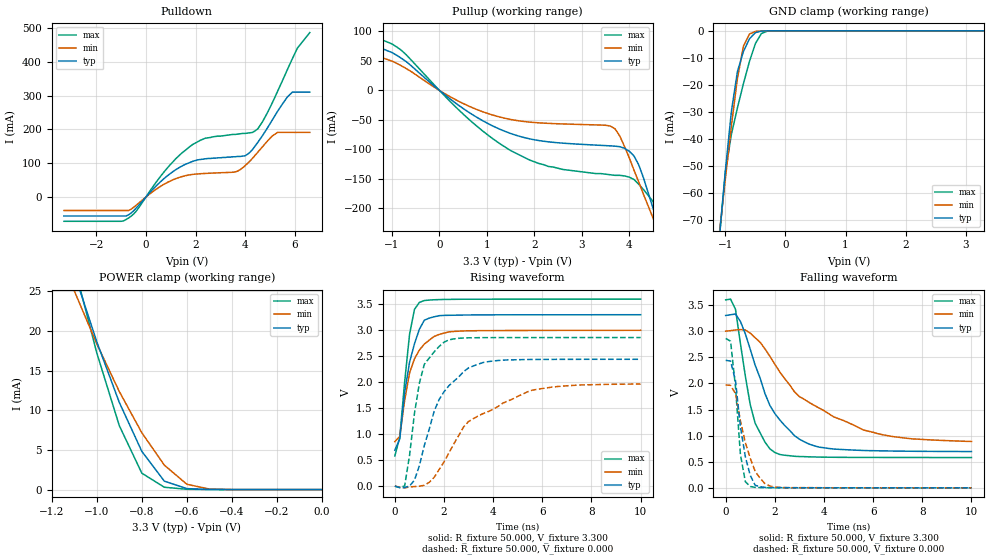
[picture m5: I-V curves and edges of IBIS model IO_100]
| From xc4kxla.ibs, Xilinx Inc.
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|   Model IO_100
[Model]   IO_100
Model_type   I/O
Polarity   Non-Inverting
Enable   Active-Low
Vinl =   0.800V
Vinh =   2.000V
Vmeas =   1.650V
Cref =  50.000pF
Rref =   1.000M
Vref =  0.000V
C_comp   7.300pF   5.500pF   8.800pF
[Temperature Range]   50.000   100.000   0.000
[Voltage Range]   3.300V   3.000V   3.600V
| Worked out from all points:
|   slope of the pulldown table from 0 to 0.495 V, typ, clamps not added: 12.8 ohm
|   slope of the pullup table from 0 to 0.495 V, typ, clamps not added: 16.3 ohm
|   GND clamp passes 1 mA (typ) near -0.52 V on its own axis
|   POWER clamp passes 1 mA (typ) near -0.69 V on its own axis
|   rising waveform, R_fixture 50.000, V_fixture 3.300: 20-80 % time 558ps typ, 647ps min, 383ps max; typ from 0.693 V to 3.3 V
|   rising waveform, R_fixture 50.000, V_fixture 0.000: 20-80 % time 1.2ns typ, 2.41ns min, 577ps max; typ from 0 V to 2.44 V
|   falling waveform, R_fixture 50.000, V_fixture 3.300: 20-80 % time 1.44ns typ, 2.95ns min, 729ps max; typ from 3.3 V to 0.696 V
|   falling waveform, R_fixture 50.000, V_fixture 0.000: 20-80 % time 438ps typ, 650ps min, 309ps max; typ from 2.44 V to 0.001 V
[Pulldown]
| voltage   I(typ)   I(min)   I(max)
-3.3V     -56.02mA   -39.74mA   -71.65mA
-900mV    -56.02mA   -39.74mA   -70.27mA
-400mV    -33.2mA    -24.66mA   -42.45mA
900mV     64.82mA    44.51mA    89.05mA
1.8V      103mA      66.09mA    151mA
3.6V      119mA      74.19mA    185mA
4V        122mA      93.03mA    188mA
4.5V      161mA      132mA      201mA
5.3V      253mA      191mA      312mA
5.7V      296mA      191mA      377mA
6.1V      310mA      191mA      440mA
6.6V      310mA      191mA      486mA
[Pullup]
| voltage   I(typ)   I(min)   I(max)
-3.3V     90.2mA     70.7mA     105mA
-1.9V     87mA       69.42mA    102mA
-1V       64.22mA    49.76mA    78.82mA
500mV     -30.67mA   -22.15mA   -40.1mA
1.5V      -72.97mA   -49.19mA   -102mA
2.3V      -87.2mA    -55.86mA   -129mA
3.6V      -94mA      -60.31mA   -143mA
3.8V      -95.43mA   -77.13mA   -144mA
4.1V      -111mA     -135mA     -151mA
4.5V      -199mA     -216mA     -188mA
4.7V      -250mA     -255mA     -227mA
6.6V      -645mA     -572mA     -737mA
[GND_clamp]
| voltage   I(typ)   I(min)   I(max)
-3.3V     -539mA     -461mA     -635mA
-1.1V     -76.29mA   -74.81mA   -76.3mA
-1V       -51.66mA   -54.6mA    -52.25mA
-900mV    -29.77mA   -35.09mA   -38.23mA
-800mV    -15.1mA    -17.65mA   -28.49mA
-700mV    -7.645mA   -5.66mA    -19.53mA
-600mV    -2.968mA   -1.205mA   -11.34mA
-500mV    -649uA     -202uA     -4.68mA
-400mV    -83.34uA   -28.89uA   -976uA
-300mV    -8.303uA   -3.567uA   -95.2uA
3.3V      90.25nA    487nA      4.544uA
[POWER_clamp]
| voltage   I(typ)   I(min)   I(max)
-3.3V     171mA      110mA      255mA
-1.1V     27.32mA    25.08mA    28.22mA
-1V       18.65mA    18.39mA    17.25mA
-900mV    11mA       12.37mA    8.069mA
-800mV    4.821mA    7.171mA    2.071mA
-700mV    1.064mA    3.083mA    296uA
-600mV    127uA      671uA      39.67uA
-500mV    14.7uA     70.21uA    9.223uA
0V        90.21nA    23.3nA     5.636uA
[Ramp]
| variable   typ   min   max
dV/dt_r   1.465/1.144n   1.179/2.496n   1.716/0.556n
dV/dt_f   1.563/1.390n   1.266/2.982n   1.811/0.717n
R_load = 50.000
[Rising Waveform]
R_fixture = 50.000
V_fixture = 3.300
V_fixture_min = 3.000
V_fixture_max = 3.600
L_fixture = 0.000H
C_fixture = 0.000F
| time   V(typ)   V(min)   V(max)
0s        693mV      856mV      580mV
200ps     906mV      954mV      936mV
400ps     1.805V     1.651V     2.006V
600ps     2.386V     2.179V     2.924V
800ps     2.741V     2.451V     3.403V
1ns       3.021V     2.619V     3.536V
1.2ns     3.193V     2.734V     3.572V
1.6ns     3.259V     2.88V      3.587V
2.2ns     3.288V     2.969V     3.594V
10ns      3.299V     2.999V     3.599V
[Rising Waveform]
R_fixture = 50.000
V_fixture = 0.000
V_fixture_min = 0.000
V_fixture_max = 0.000
L_fixture = 0.000H
C_fixture = 0.000F
| time   V(typ)   V(min)   V(max)
0s        0V         0V         0V
400ps     -27.04mV   -33.2mV    4.185mV
800ps     115mV      -8.135mV   1.403V
1ns       395mV      -1.755mV   1.984V
1.2ns     782mV      17.29mV    2.344V
1.6ns     1.441V     169mV      2.583V
2ns       1.815V     466mV      2.77V
3ns       2.276V     1.244V     2.855V
5.4ns     2.437V     1.816V     2.859V
10ns      2.441V     1.965V     2.86V
[Falling Waveform]
R_fixture = 50.000
V_fixture = 3.300
V_fixture_min = 3.000
V_fixture_max = 3.600
L_fixture = 0.000H
C_fixture = 0.000F
| time   V(typ)   V(min)   V(max)
0s        3.3V       3V         3.599V
200ps     3.314V     3.009V     3.613V
400ps     3.328V     3.023V     3.418V
1ns       2.654V     2.963V     1.594V
1.2ns     2.349V     2.874V     1.238V
2ns       1.424V     2.368V     678mV
2.8ns     1V         1.838V     605mV
3.4ns     837mV      1.634V     594mV
5.6ns     716mV      1.109V     583mV
10ns      696mV      889mV      581mV
[Falling Waveform]
R_fixture = 50.000
V_fixture = 0.000
V_fixture_min = 0.000
V_fixture_max = 0.000
L_fixture = 0.000H
C_fixture = 0.000F
| time   V(typ)   V(min)   V(max)
0s        2.442V     1.97V      2.861V
200ps     2.426V     1.963V     2.808V
400ps     2.055V     1.805V     1.932V
600ps     1.173V     1.286V     644mV
800ps     598mV      870mV      119mV
1ns       239mV      568mV      27.26mV
1.2ns     49.64mV    318mV      9.389mV
1.4ns     23.1mV     184mV      6.819mV
2ns       6.438mV    16.07mV    2.998mV
10ns      647uV      831uV      496uV
